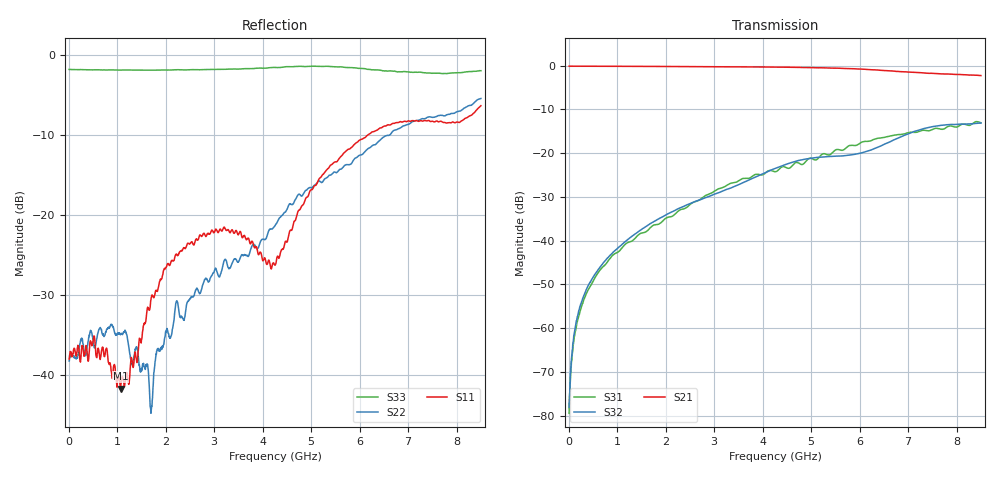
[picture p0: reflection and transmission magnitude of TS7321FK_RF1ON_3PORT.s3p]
!Created with skrf (http://scikit-rf.org).
# GHz S RI R 50.0
!freq ReS11 ImS11 ReS12 ImS12 ReS13 ImS13
! ReS21 ImS21 ReS22 ImS22 ReS23 ImS23
! ReS31 ImS31 ReS32 ImS32 ReS33 ImS33
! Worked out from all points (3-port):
!   1601 points, 10 MHz to 8.5 GHz, reference 50 ohm
!   strongest paths, dB at 10 MHz, 2.132 GHz, 4.255 GHz, 6.378 GHz, 8.5 GHz:
!     S21: -0.1, -0.2, -0.4, -1.0, -2.3
!     S32: -78.2, -33.4, -23.5, -18.7, -13.2
!     S31: -79.5, -34.5, -24.3, -16.6, -13.1
!   lowest |S11| = -41.6 dB at 1.071 GHz (marker M1), VSWR 1.02, Z = 50.8 + j0.171 ohm
!   |S11| at or under -10 dB: start of sweep to 6.162 GHz
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0.01  0.0127 4.63e-07  0.9835 -0.00447  5.86e-05 4.08e-05
      0.9835 -0.00451  0.0121 0.00231  6.58e-05 9.53e-05
      5.9e-05 8.8e-05  0.00011 5.55e-05  -0.8132 0.00401
0.1002062  0.0143 0.00229  0.982 -0.0304  8.83e-05 0.000668
           0.9824 -0.0306  0.013 0.00101  8.38e-05 0.000742
           7.62e-05 0.000685  9.61e-05 0.000733  -0.8107 0.0356
0.2753125  0.0137 0.0069  0.9782 -0.0834  -3.68e-05 0.00181
           0.9783 -0.0834  0.0161 0.0053  8.91e-05 0.00207
           -2.57e-05 0.00184  9.03e-05 0.00204  -0.8052 0.0949
1.07125  0.0081 0.00168  0.9281 -0.316  -0.00107 0.00782
         0.9276 -0.3157  0.0175 0.00475  2.99e-05 0.00874
         -0.00107 0.00781  5.18e-05 0.00874  -0.7267 0.3471
1.702694  0.00674 -0.0298  0.847 -0.4883  -0.0022 0.0142
          0.847 -0.4881  0.00233 -0.00561  0.00108 0.0158
          -0.00222 0.0141  0.00111 0.0158  -0.6154 0.5185
2.222706  0.00887 -0.0566  0.7544 -0.6163  -0.00341 0.0205
          0.7544 -0.6159  -0.0258 -0.0133  0.00359 0.0223
          -0.00344 0.0205  0.00358 0.0223  -0.4968 0.6399
3.225588  0.0477 -0.0676  0.5243 -0.8127  0.00188 0.0414
          0.5248 -0.8128  -0.0372 0.0378  0.0128 0.0355
          0.00183 0.0414  0.0129 0.0356  -0.2355 0.7804
4.255  -0.0108 -0.0475  0.2282 -0.9324  0.0222 0.057
       0.2288 -0.932  -0.0601 0.0615  0.0378 0.0548
       0.0221 0.057  0.0378 0.0547  0.0573 0.834
5.958306  -0.2817 -0.0541  -0.2998 -0.8625  0.0784 0.0965
          -0.2997 -0.8625  -0.0951 0.2116  0.0908 0.0372
          0.0784 0.0966  0.0909 0.0372  0.397 0.7269
8.5  -0.2854 0.3891  -0.742 -0.2032  0.2134 -0.0597
     -0.7404 -0.2035  0.2741 0.4597  0.1585 -0.1526
     0.213 -0.0594  0.1582 -0.1529  0.7687 0.2156
